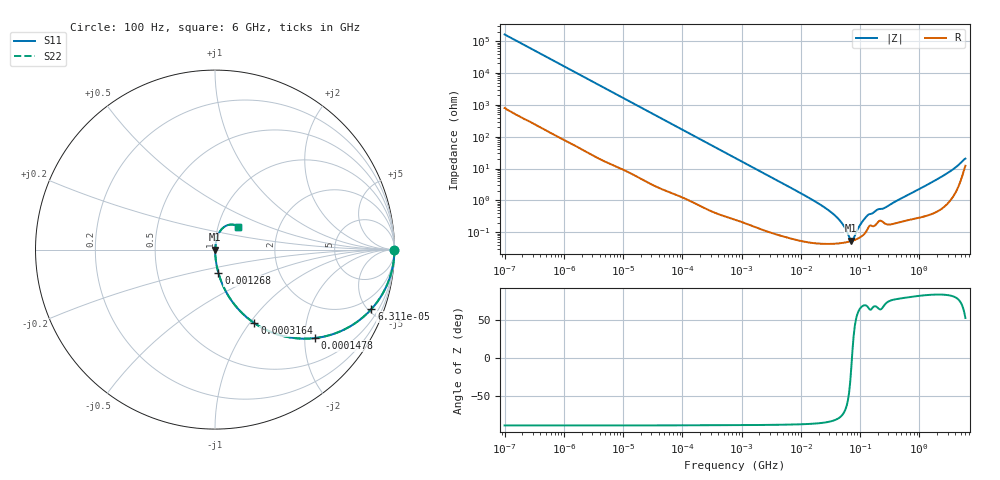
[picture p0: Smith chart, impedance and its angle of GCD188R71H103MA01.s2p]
!Murata Part Number: GCD188R71H103MA01
!These Parameters are Measured in Series Mode Connection
!Data Generated on Mar 13, 2026
!  o--ll--o
!Port1  Port2
!  o------o
!Operation Temp=25[degC], DC Bias Voltage=0[V]
!Freq. Start=100[Hz] Stop=6[GHz] 401[Steps]
# Hz S RI R 50
!Freq.(Hz) S11(Real) S11(Imag) S21(Real) S21(Imag) S12(Real) S12(Imag) S22(Real) S22(Imag)
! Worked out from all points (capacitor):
!   401 points, 100 Hz to 6 GHz, reference 50 ohm
!   read as one part in series: C = 9.8 nF near 109 Hz
!   lowest |Z| = 54.1 mohm at 71.29 MHz (marker M1)
!   series resonance near 73 MHz, so ESL is about 490 pH
!   S11 on the Smith chart (normalised r, x): 100 Hz: open; 63.12 kHz: 1.04, -5.25; 147.8 kHz: 1.02, -2.25; 316.4 kHz: 1.01, -1.05; 1.268 MHz: 1.00, -0.27; 6 GHz: 1.25, +0.33
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100  1 -0.000616  3.4e-06 0.000616  3.4e-06 0.000616  1 -0.000616
2008  0.9998 -0.0123  0.000211 0.0123  0.000211 0.0123  0.9998 -0.0123
12041  0.9943 -0.0727  0.00573 0.0727  0.00573 0.0727  0.9943 -0.0727
40335  0.9426 -0.2296  0.0574 0.2296  0.0574 0.2296  0.9426 -0.2296
63115  0.8715 -0.3313  0.1285 0.3313  0.1285 0.3313  0.8715 -0.3313
147774  0.5584 -0.4927  0.4416 0.4927  0.4416 0.4927  0.5584 -0.4927
316350  0.2196 -0.4098  0.7804 0.4098  0.7804 0.4098  0.2196 -0.4098
774597  0.0469 -0.2057  0.9531 0.2057  0.9531 0.2057  0.0469 -0.2057
1267578  0.019 -0.1299  0.981 0.1299  0.981 0.1299  0.019 -0.1299
3549919  0.00316 -0.0475  0.9968 0.0475  0.9968 0.0475  0.00316 -0.0475
1.555665e7  0.000572 -0.0105  0.9994 0.0105  0.9994 0.0105  0.000572 -0.0105
2.784235e7  0.000458 -0.00527  0.9995 0.00527  0.9995 0.00527  0.000458 -0.00527
3.983537e7  0.000449 -0.00303  0.9996 0.00303  0.9996 0.00303  0.000449 -0.00303
5.211241e7  0.000469 -0.00162  0.9995 0.00162  0.9995 0.00162  0.000469 -0.00162
6.518806e7  0.000507 -0.000536  0.9995 0.000536  0.9995 0.000536  0.000507 -0.000536
7.129496e7  0.00053 -0.000111  0.9995 0.000111  0.9995 0.000111  0.00053 -0.000111
7.797396e7  0.000559 0.000315  0.9994 -0.000315  0.9994 -0.000315  0.000559 0.000315
1.020051e8  0.000709 0.00165  0.9993 -0.00165  0.9993 -0.00165  0.000709 0.00165
1.334425e8  0.00125 0.00314  0.9988 -0.00314  0.9988 -0.00314  0.00125 0.00314
3.124326e8  0.0018 0.00692  0.9982 -0.00692  0.9982 -0.00692  0.0018 0.00692
3.352442e9  0.0165 0.0802  0.9835 -0.0802  0.9835 -0.0802  0.0165 0.0802
6e9  0.128 0.128  0.872 -0.128  0.872 -0.128  0.128 0.128
